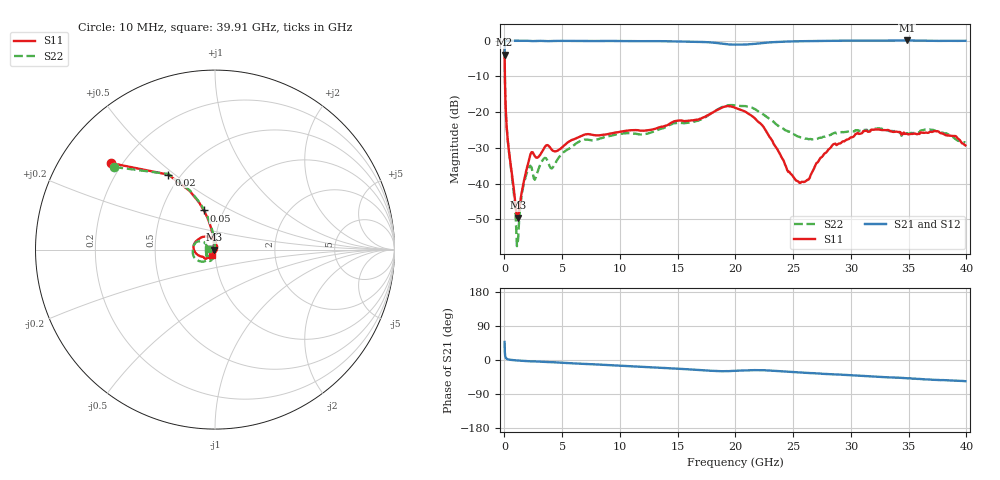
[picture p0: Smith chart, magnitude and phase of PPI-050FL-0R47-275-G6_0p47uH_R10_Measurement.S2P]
! Data measured by Modelithics Inc.  support@modelithics.com  813-866-6335  Tampa FL USA June 2025
! PPI-050FL-0R47-275-G6_0p47uH measured on 10-mil thick RO4350B board, mounted in 2-port shunt configuration on a 50-ohm transmission line
# Hz S MA R 50
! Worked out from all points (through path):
!   429 points, 10 MHz to 39.91 GHz, reference 50 ohm
!   highest |S21| = 0.05 dB at 34.86 GHz (marker M1); lowest = -3.9 dB at 10 MHz (marker M2)
!   group delay of S21, straight-line fit = 3.92 ps
!   lowest |S11| = -49.6 dB at 1.174 GHz (marker M3), VSWR 1.01, Z = 49.7 - j0.0942 ohm
!   |S11| at or under -10 dB: 34.78 MHz to end of sweep
!   |S22| runs from -57.5 to -2.8 dB; largest |S21 - S12| = 0.025
!   S11 on the Smith chart (normalised r, x): 10 MHz: 0.16, +0.35; 20 MHz: 0.43, +0.47; 50 MHz: 0.81, +0.37; 39.91 GHz: 0.96, -0.06
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1e7  0.7547 140.3  0.6383 47.6  0.6382 47.6  0.7251 140.6
2e7  0.4916 121.9  0.8518 29.5  0.8518 29.5  0.4944 121.6
5e7  0.2268 105.8  0.9648 13.0  0.9648 13.0  0.2266 105.1
2e8  0.05867 98.1  0.995 3.1  0.9951 3.1  0.05856 95.1
9.796215e8  0.004519 135.7  0.9979 -0.9  0.998 -0.9  0.003179 106.0
1.173799e9  0.003309 -163.4  0.9979 -1.4  0.998 -1.4  0.001622 -140.9
1.659243e9  0.0104 -106.9  0.9973 -2.4  0.9974 -2.4  0.009634 -108.7
2.144687e9  0.02239 -106.2  0.9922 -3.5  0.9924 -3.5  0.01726 -122.4
2.72722e9  0.02307 -128.4  0.9905 -3.9  0.9907 -3.9  0.01235 -113.6
3.406841e9  0.03079 -118.9  0.9892 -5.2  0.9894 -5.3  0.02233 -113.7
4.183552e9  0.0288 -132.4  0.9883 -5.9  0.9885 -5.9  0.01679 -106.2
6.70786e9  0.0467 -116.6  0.9891 -10.1  0.9892 -10.0  0.04026 -99.6
1.340699e10  0.06114 -132.0  0.9835 -20.4  0.9837 -20.4  0.05735 -107.2
2.000902e10  0.1143 154.6  0.8786 -28.3  0.8788 -28.4  0.1241 -176.2
2.233916e10  0.06482 101.8  0.9229 -26.8  0.9231 -27.0  0.09456 149.9
2.534891e10  0.01085 7.3  0.9783 -32.5  0.9785 -32.2  0.04597 158.8
2.670815e10  0.01505 -86.4  0.9865 -34.7  0.9867 -34.7  0.04161 178.0
2.845575e10  0.03517 -115.0  0.9952 -37.8  0.9954 -37.4  0.05028 -160.1
3.331019e10  0.05517 -116.1  1.001 -45.7  1.002 -45.8  0.05416 -141.3
3.486361e10  0.04942 -117.8  1.006 -47.9  1.006 -48.9  0.05075 -133.3
3.738792e10  0.05396 -120.7  0.9913 -52.4  0.9914 -52.0  0.05402 -154.6
3.991223e10  0.03411 -120.3  0.9942 -56.0  0.9944 -55.4  0.03748 175.8
